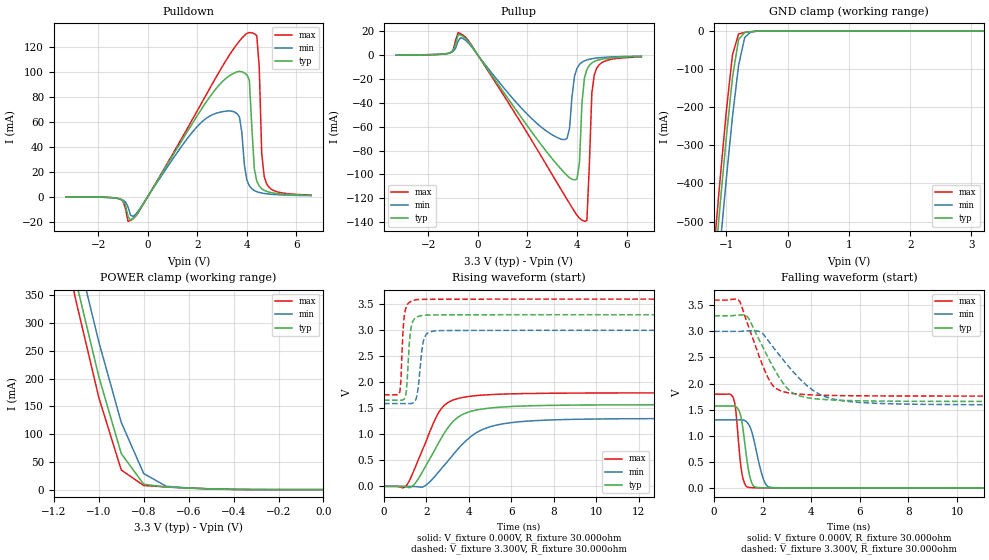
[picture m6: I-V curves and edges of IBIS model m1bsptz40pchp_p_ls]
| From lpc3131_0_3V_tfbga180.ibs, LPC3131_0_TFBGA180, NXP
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| |   Rev 0.20 IBIS Model Design Automation Generation   |
| |   N O N - S I L I C O N   C O R R E L A T E D   |
| |   This IBIS [Model] is pre-Beta tactical support   |
| |  Note: this IBIS [Model] contains clamp curves generated   |
| |   through simulation which should not be relied upon   |
| Date/Time   : 2010 Jan 25 (Mon) 11:58:19
| Pccmos090 jliolib_p50 2.0
|   0.9 um 3.3V pad library
|   seven level metal
|   dual oxide
|   dual threshold voltage
|   nominal line mixed supply
|   parasitic extracted netlists
| Process block a10
| mem1bsptz40pchp
|   Bidirectional Pad 3.3
|   3state Output
|   Plain Input
|   CMOS
|   Programmable between
|   - (p1=0, p2=1) plain input
|   - (p1=0, p2=0) with Pull Up
|   - (p1=1, p2=1) with Pull Down
|   - (p1=1, p2=0) with Repeater
| Plain input Mode low speed (esh=1, p1=0, p2=1)
[Model]   m1bsptz40pchp_p_ls | of mem1bsptz40pchp
Model_type   I/O
Polarity   Non-Inverting
Enable   Active-Low
|  Reciever Thresholds
Vinl   = 0.99V
Vinh   = 2.31V
| AC Test Load Conditions
Vref   = 0
Cref   = 0
Rref   = 1000000000
Vmeas   = 1.65
| [Process Range]   typical   min   max
| C_comp edge width   400.000ps   400.000ps   400.000ps
| C_comp Tstrobe   40.000fs   40.000fs   40.000fs
C_comp   200.000pF   200.000pF   200.000pF
[Temperature Range]   25   125   -40
[Voltage Range]   3.30V   3.00V   3.60V
[GND Clamp Reference]   0.00V   0.00V   0.00V
[Pulldown Reference]   0.00V   0.00V   0.00V
[POWER Clamp Reference]   3.30V   3.00V   3.60V
[Pullup Reference]   3.30V   3.00V   3.60V
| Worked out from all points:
|   slope of the pulldown table from 0 to 0.495 V, typ, clamps not added: 30.7 ohm
|   slope of the pullup table from 0 to 0.495 V, typ, clamps not added: 33.2 ohm
|   GND clamp passes 1 mA (typ) near -0.52 V on its own axis
|   POWER clamp passes 1 mA (typ) near -0.48 V on its own axis
|   rising waveform, V_fixture 0.000V, R_fixture 30.000ohm: 20-80 % time 1.41ns typ, 1.86ns min, 1.14ns max; typ from 0 V to 1.57 V
|   falling waveform, V_fixture 0.000V, R_fixture 30.000ohm: 20-80 % time 278ps typ, 397ps min, 215ps max; typ from 1.57 V to 0 V
|   rising waveform, V_fixture 3.300V, R_fixture 30.000ohm: 20-80 % time 164ps typ, 222ps min, 138ps max; typ from 1.66 V to 3.3 V
|   falling waveform, V_fixture 3.300V, R_fixture 30.000ohm: 20-80 % time 1.16ns typ, 1.67ns min, 890ps max; typ from 3.3 V to 1.66 V
[GND Clamp]
| ref voltage   0.00V   0.00V   0.00V
|   Voltage   I(typ)   I(min)   I(max)
-3.3V     -4.732A    -4.814A    -4.684A
-1.2V     -636mA     -742.5mA   -569.7mA
-1.1V     -453.5mA   -561.8mA   -385.7mA
-1V       -279mA     -387.5mA   -210.8mA
-900mV    -122.8mA   -225.5mA   -63.11mA
-800mV    -22.42mA   -90.48mA   -8.158mA
-700mV    -4.346mA   -17.29mA   -4.479mA
-600mV    -2.103mA   -3.017mA   -2.46mA
-300mV    -3.346uA   -19.56uA   -987.1nA
3.2V      182pA      6.98uA     191.9pA
[Power Clamp]   | Vtable = Vcc - Vpad
| ref voltage   3.30V   3.00V   3.60V
|   Voltage   I(typ)   I(min)   I(max)
-3.3V     4.647A     4.675A     4.636A
-1.2V     553.3mA    610.4mA    520.8mA
-1.1V     373.2mA    433.6mA    337.9mA
-1V       204mA      266.6mA    166.4mA
-900mV    65.06mA    121.2mA    35.38mA
-800mV    9.603mA    28.92mA    7.422mA
-700mV    4.54mA     6.054mA    4.861mA
-600mV    2.669mA    2.794mA    2.852mA
-400mV    308.1uA    509.7uA    227.2uA
0V        393.8pA    9.961nA    269.9pA
[Pulldown]
| ref voltage   0.00V   0.00V   0.00V
|   Voltage   I(typ)   I(min)   I(max)
-3.3V     -236.8uA   -252.6uA   -192.2uA
-1.2V     -1.654mA   -1.557mA   -1.498mA
-600mV    -17.59mA   -16.04mA   -17.81mA
2.9V      89.68mA    67.41mA    100.4mA
3.7V      100.2mA    63.84mA    124.5mA
4.1V      93.21mA    8.525mA    131.3mA
4.3V      22.46mA    4.748mA    130.4mA
4.4V      12.41mA    3.864mA    128.9mA
4.5V      8.379mA    3.247mA    103.7mA
4.6V      6.229mA    2.794mA    34.8mA
4.8V      4.116mA    2.178mA    10.07mA
6.6V      977.1uA    710.9uA    1.218mA
[Pullup]   | Vtable = Vcc - Vpad
| ref voltage   3.30V   3.00V   3.60V
|   Voltage   I(typ)   I(min)   I(max)
-3.3V     206.9uA    209uA      174.2uA
-500mV    14.09mA    12.45mA    15.05mA
3.4V      -96.53mA   -70.69mA   -114.1mA
3.7V      -102.8mA   -61.23mA   -124.3mA
3.9V      -104.5mA   -17.63mA   -131mA
4.1V      -90.2mA    -7.678mA   -136.7mA
4.2V      -40.59mA   -5.874mA   -138.2mA
4.3V      -19.19mA   -4.731mA   -139.3mA
4.4V      -11.92mA   -3.949mA   -138.6mA
4.6V      -6.518mA   -2.953mA   -31.79mA
4.7V      -5.293mA   -2.618mA   -16.38mA
6.6V      -1.121mA   -811.2uA   -1.417mA
[Ramp]
R_load   = 30.000ohm
|   dV/dt(typ)   dV/dt(min)   dV/dt(max)
dV/dt_r   941.604mV/1.400ns   782.818mV/1.900ns   1.078V/1.150ns
dV/dt_f   986.365mV/1.150ns   844.768mV/1.700ns   1.104V/900.000ps
[Rising Waveform]  | cubic spline decimation from 501 points
V_fixture   = 0.000V
R_fixture   = 30.000ohm
|   Time   V(typ)   V(min)   V(max)
0s        4.028nV    182.8nV    2.848nV
950ps     -5.394mV   33.04uV    -20.27mV
1.35ns    8.492mV    -1.864mV   245.6mV
1.85ns    306.6mV    -8.845mV   734.8mV
2.6ns     855.7mV    288.5mV    1.433V
3.15ns    1.199V     555.4mV    1.641V
3.75ns    1.391V     832mV      1.713V
5ns       1.506V     1.147V     1.763V
7.15ns    1.552V     1.264V     1.787V
25ns      1.569V     1.305V     1.797V
[Falling Waveform]  | cubic spline decimation from 501 points
V_fixture   = 0.000V
R_fixture   = 30.000ohm
|   Time   V(typ)   V(min)   V(max)
0s        1.569V     1.305V     1.797V
800ps     1.57V      1.305V     1.715V
900ps     1.556V     1.305V     1.458V
1.05ns    1.455V     1.305V     642.5mV
1.15ns    1.256V     1.305V     262.3mV
1.45ns    260.6mV    1.195V     7.533mV
1.65ns    25.89mV    897.6mV    2.146mV
2ns       2.484mV    211mV      854.9uV
2.35ns    965.4uV    8.802mV    595.7uV
25ns      22.06nV    233.6nV    26.61nV
[Rising Waveform]  | cubic spline decimation from 501 points
V_fixture   = 3.300V
V_fixture_min = 3.000V
V_fixture_max = 3.600V
R_fixture   = 30.000ohm
|   Time   V(typ)   V(min)   V(max)
0s        1.656V     1.592V     1.76V
750ps     1.656V     1.592V     1.819V
800ps     1.656V     1.592V     2.044V
900ps     1.663V     1.592V     3.015V
1ns       1.713V     1.592V     3.378V
1.25ns    2.982V     1.592V     3.552V
1.5ns     3.246V     1.669V     3.587V
1.85ns    3.289V     2.778V     3.596V
2.35ns    3.296V     2.986V     3.598V
25ns      3.3V       3V         3.6V
[Falling Waveform]  | cubic spline decimation from 501 points
V_fixture   = 3.300V
V_fixture_min = 3.000V
V_fixture_max = 3.600V
R_fixture   = 30.000ohm
|   Time   V(typ)   V(min)   V(max)
0s        3.3V       3V         3.6V
1ns       3.313V     3V         3.604V
1.35ns    3.291V     3.01V      3.182V
1.9ns     2.798V     2.989V     2.467V
2.3ns     2.429V     2.777V     2.043V
2.55ns    2.219V     2.627V     1.907V
3.1ns     1.87V      2.31V      1.819V
4.4ns     1.699V     1.781V     1.776V
6.05ns    1.669V     1.636V     1.765V
25ns      1.656V     1.592V     1.76V
